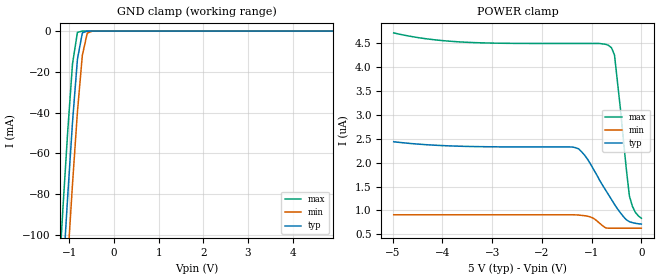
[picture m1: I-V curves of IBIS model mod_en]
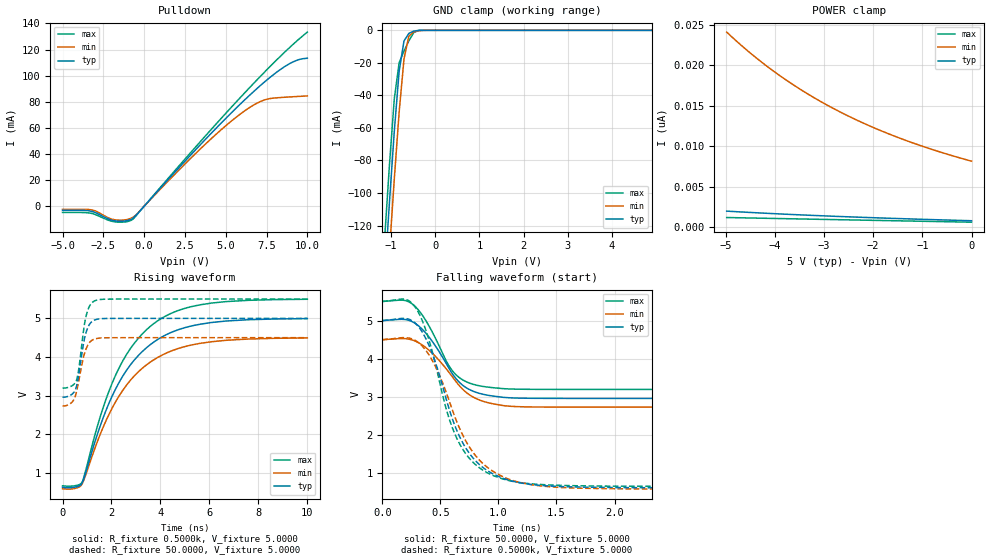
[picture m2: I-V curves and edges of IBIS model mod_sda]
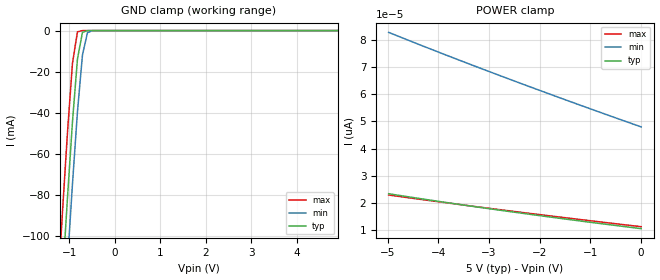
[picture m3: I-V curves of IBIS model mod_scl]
| IBIS (I/O, Buffer, Information, Specification) Model, officially
| electronic behavioral standard for Buffer structures of digital pins.
[IBIS ver]  4.0
[File name] m24c04_fa3_tssop8.ibs
[File Rev]  1.0
[Date]   5 Dic 2014
[Source]   CAD & Design Services (Catania) - STMicroelectronics
[Notes]
   (Note1)  This IBIS model includes the TSSOP8 package data
   (Note2)  This IBIS model has some Notes about the non-monotonicity
   of the I-V curves, but they are not indicative of problems
   inside the model;
[Copyright] (c) 2014 STMicroelectronics
|   Component M24C04
[Component] M24C04
[Manufacturer] STMicroelectronics
[Package]
| variable   typ   min   max
R_pkg   0.0   0.0   0.0
L_pkg   0.0H   0.0H   0.0H
C_pkg   0.0F   0.0F   0.0F
[Pin]  signal_name   model_name   R_pin   L_pin   C_pin
1   NC   NC   NA   NA   NA
2   E1   mod_en   NA   NA   NA
3   E2   mod_en   NA   NA   NA
4   VSS   GND   NA   NA   NA
5   SDA   mod_sda   NA   NA   NA
6   SCL   mod_scl   NA   NA   NA
7   WCN   mod_wc   NA   NA   NA
8   VCC   POWER   NA   NA   NA
[Package Model]  182696_TSSOP8
[Define Package Model]  182696_TSSOP8
[Manufacturer]  STMicroelectronics
[OEM]  STMicroelectronics
[Description]  8 pin TSSOP package
[Number Of Pins]  8
[Pin Numbers]
|Pin Num   Terminal Name
1   | net1
2   | net2
3   | net3
4   | net4_GND
5   | net5
6   | net6
7   | net7
8   | net8_VDD
[Model Data]
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[End Model Data]
[End Package Model]
| Models and submodels in the file (4): mod_en (Input), mod_sda (I/O_open_drain), mod_scl (Input), mod_wc (Input)
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|   Model mod_en
[Model]   mod_en
Model_type Input
Vinl   =   1.500V
Vinh   =   3.500V
C_comp   1.763pF   1.683pF   1.933pF
[Temperature Range]   25.0000   85.0000   -40.0000
[Voltage Range]   5.0000V   4.5000V   5.5000V
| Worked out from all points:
|   GND clamp passes 1 mA (typ) near -0.71 V on its own axis
[GND_clamp]
|Voltage   I(typ)   I(min)   I(max)
-5V       -1.63A     -1.659A    -1.601A
-1.26V    -162.1mA   -194mA     -129.6mA
-1.15V    -121.4mA   -153.3mA   -88.92mA
-1.04V    -81.84mA   -113.4mA   -50.02mA
-930mV    -44.68mA   -75mA      -16.05mA
-820mV    -13.86mA   -39.64mA   -620.3uA
-710mV    -876.1uA   -11.9mA    -4.426uA
-600mV    -18.76uA   -1.022mA   -29.45nA
-490mV    -372.8nA   -42.05uA   -196.9pA
4.9V      10.41pA    50.62pA    10.07pA
[POWER_clamp]
|Voltage   I(typ)   I(min)   I(max)
-4.98V    2.436uA    909.7nA    4.711uA
-3.66V    2.343uA    909.7nA    4.523uA
-1.32V    2.31uA     907.6nA    4.49uA
-1.08V    2.067uA    880nA      4.49uA
-660mV    1.327uA    630.1nA    4.45uA
-600mV    1.227uA    630.1nA    4.399uA
-540mV    1.127uA    630.1nA    4.247uA
-420mV    950nA      630.1nA    3.114uA
-300mV    803.3nA    630.1nA    1.84uA
-240mV    766.1nA    630.1nA    1.299uA
-120mV    732.1nA    630.1nA    959.6nA
0V        716.8nA    630.1nA    837nA
|   Model mod_sda
[Model]   mod_sda
Model_type I/O_open_drain
Polarity   Non-Inverting
Vinl   =   1.500V
Vinh   =   3.500V
Vmeas  =   2.500V
Cref   =   10pF
Rref   =   1k
Vref   =   5.000V
C_comp   3.856pF   3.682pF   4.038pF
[Temperature Range]  25.0000   85.0000   -40.0000
[Voltage Range]   5.0000V   4.5000V   5.5000V
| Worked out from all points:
|   slope of the pulldown table from 0 to 0.75 V, typ, clamps not added: 71.5 ohm
|   GND clamp passes 1 mA (typ) near -0.53 V on its own axis
|   rising waveform, R_fixture 0.5000k, V_fixture 5.0000: 20-80 % time 2.05ns typ, 2.09ns min, 1.98ns max; typ from 0.625 V to 4.99 V
|   rising waveform, R_fixture 50.0000, V_fixture 5.0000: 20-80 % time 326ps typ, 359ps min, 299ps max; typ from 2.96 V to 5 V
|   falling waveform, R_fixture 50.0000, V_fixture 5.0000: 20-80 % time 272ps typ, 307ps min, 244ps max; typ from 5 V to 2.96 V
|   falling waveform, R_fixture 0.5000k, V_fixture 5.0000: 20-80 % time 325ps typ, 360ps min, 295ps max; typ from 5 V to 0.625 V
[Pulldown]
|Voltage   I(typ)   I(min)   I(max)
-5V       -3.143mA   -2.328mA   -4.707mA
-3.24V    -3.798mA   -2.726mA   -5.388mA
-1.64V    -11.41mA   -10.63mA   -12.13mA
-1V       -10.86mA   -10.02mA   -11.64mA
-680mV    -9.205mA   -8.463mA   -9.861mA
3.48V     47.6mA     44.34mA    50mA
4.92V     66.24mA    60.77mA    70.04mA
6.2V      81.94mA    73.41mA    87.37mA
7.32V     94.61mA    81.22mA    102mA
8.6V      106.9mA    83.49mA    117.9mA
9.4V      112mA      84.09mA    127.1mA
10V       113.4mA    84.5mA     133.4mA
[GND_clamp]
|Voltage   I(typ)   I(min)   I(max)
-5V       -1.909A    -1.935A    -1.889A
-1.15V    -152.1mA   -182.6mA   -128.8mA
-1.04V    -105.9mA   -136.2mA   -82.98mA
-930mV    -62.22mA   -91.56mA   -42.15mA
-820mV    -25.14mA   -50.33mA   -19.97mA
-710mV    -6.551mA   -17.64mA   -12.75mA
-600mV    -1.891mA   -3.57mA    -6.485mA
-490mV    -473.2uA   -1.038mA   -1.394mA
-380mV    -44.76uA   -237.8uA   -20.03uA
4.9V      782.5pA    8.841nA    551.8pA
[POWER_clamp]
|Voltage   I(typ)   I(min)   I(max)
-4.98V    1.985nA    24.08nA    1.196nA
-4.74V    1.901nA    22.75nA    1.168nA
-4.44V    1.803nA    21.2nA     1.132nA
-3.9V     1.639nA    18.71nA    1.068nA
-3.36V    1.491nA    16.56nA    1.005nA
-2.76V    1.343nA    14.5nA     935pA
-2.16V    1.207nA    12.74nA    865.8pA
-1.5V     1.071nA    11.09nA    790.2pA
-780mV    935.4pA    9.555nA    708.2pA
0V        799.3pA    8.15nA     619.7pA
[Ramp]
| variable   typ   min   max
dV/dt_r   1.2220/0.3742n   1.0587/0.4127n   1.3808/0.3408n
dV/dt_f   1.2220/0.2985n   1.0587/0.3332n   1.3200/0.3440n
R_load = 50.0000
[Rising Waveform]
R_fixture= 0.5000k
V_fixture= 5.0000
V_fixture_min= 4.5000
V_fixture_max= 5.5000
|time   V(typ)   V(min)   V(max)
0s        625.5mV    590mV      664.1mV
480ps     627mV      593mV      664.3mV
800ps     735.2mV    712.6mV    758.2mV
1.56ns    2.252V     2.031V     2.493V
2.18ns    3.186V     2.853V     3.545V
2.94ns    3.928V     3.517V     4.362V
3.74ns    4.393V     3.932V     4.871V
4.54ns    4.663V     4.179V     5.158V
5.63ns    4.85V      4.354V     5.352V
10ns      4.994V     4.494V     5.495V
[Rising Waveform]
R_fixture= 50.0000
V_fixture= 5.0000
V_fixture_min= 4.5000
V_fixture_max= 5.5000
|time   V(typ)   V(min)   V(max)
0s        2.963V     2.735V     3.199V
380ps     3.034V     2.827V     3.253V
480ps     3.099V     2.918V     3.302V
560ps     3.216V     3.074V     3.381V
660ps     3.53V      3.368V     3.674V
860ps     4.357V     4.003V     4.693V
960ps     4.633V     4.209V     5.052V
1.12ns    4.862V     4.388V     5.337V
1.36ns    4.969V     4.474V     5.465V
10ns      5V         4.5V       5.5V
[Falling Waveform]
R_fixture= 50.0000
V_fixture= 5.0000
V_fixture_min= 4.5000
V_fixture_max= 5.5000
|time   V(typ)   V(min)   V(max)
0s        5V         4.5V       5.5V
190ps     5.03V      4.529V     5.528V
290ps     4.912V     4.454V     5.346V
410ps     4.538V     4.203V     4.815V
570ps     3.774V     3.661V     3.835V
670ps     3.365V     3.273V     3.492V
810ps     3.12V      2.957V     3.311V
1.03ns    2.996V     2.782V     3.223V
1.53ns    2.965V     2.737V     3.2V
10ns      2.963V     2.735V     3.199V
[Falling Waveform]
R_fixture= 0.5000k
V_fixture= 5.0000
V_fixture_min= 4.5000
V_fixture_max= 5.5000
|time   V(typ)   V(min)   V(max)
0s        5V         4.5V       5.5V
190ps     5.058V     4.555V     5.56V
300ps     4.882V     4.449V     5.273V
420ps     4.215V     4.011V     4.301V
580ps     2.64V      2.863V     2.392V
720ps     1.659V     1.844V     1.51V
900ps     1.084V     1.171V     1.026V
1.16ns    771.8mV    785.2mV    774.1mV
2.16ns    629.7mV    597.4mV    666.2mV
10ns      625.5mV    590mV      664.1mV
|   Model mod_scl
[Model]   mod_scl
Model_type Input
Vinl   =   1.500V
Vinh   =   3.500V
C_comp   1.763pF   1.683pF   1.933pF
[Temperature Range]  25.0000   85.0000   -40.0000
[Voltage Range]   5.0000V   4.5000V   5.5000V
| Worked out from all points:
|   GND clamp passes 1 mA (typ) near -0.71 V on its own axis
[GND_clamp]
|Voltage   I(typ)   I(min)   I(max)
-5V       -1.63A     -1.659A    -1.601A
-1.26V    -162.1mA   -194mA     -129.6mA
-1.15V    -121.4mA   -153.3mA   -88.92mA
-1.04V    -81.84mA   -113.4mA   -50.02mA
-930mV    -44.68mA   -75mA      -16.05mA
-820mV    -13.86mA   -39.64mA   -620.3uA
-710mV    -876.1uA   -11.9mA    -4.426uA
-600mV    -18.76uA   -1.022mA   -29.45nA
-490mV    -372.8nA   -42.05uA   -196.9pA
4.9V      10.41pA    50.62pA    10.07pA
[POWER_clamp]
|Voltage   I(typ)   I(min)   I(max)
-4.98V    23.46pA    82.67pA    22.99pA
-3.78V    20.06pA    73.87pA    19.99pA
-2.58V    16.89pA    65.38pA    17.13pA
-1.32V    13.75pA    56.76pA    14.26pA
0V        10.64pA    47.99pA    11.36pA
